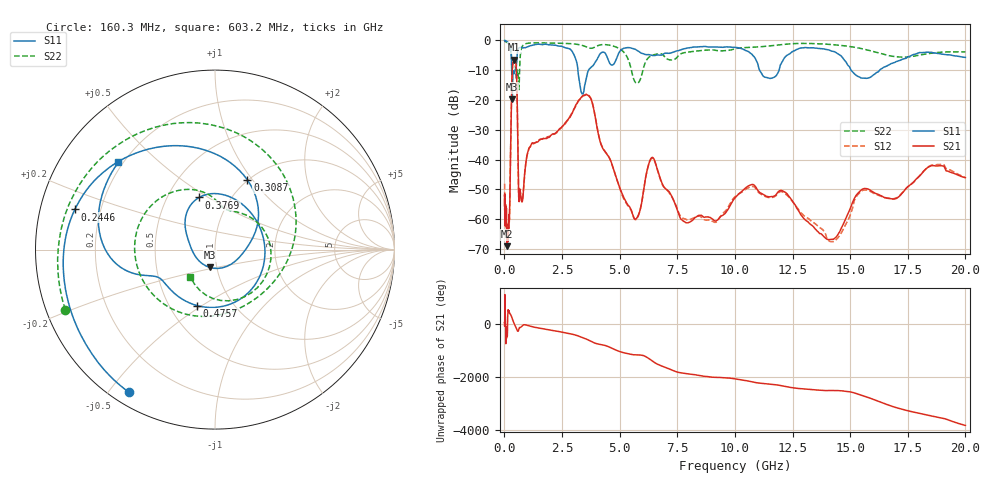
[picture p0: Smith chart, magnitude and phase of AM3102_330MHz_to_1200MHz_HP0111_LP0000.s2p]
! Date/Time: Tue, Sep 11, 2018 5:15 PM
! Network Analyzer: Agilent Technologies E8362B Rev: A.07.50.63
! Sweep from 0.010 to 20.000 GHz, 1601 Points, Sweep Type: LOG
! Power Supply: 4.949 V, 0.001 A
# Hz S DB R 50
!freq MagS11 AngS11 MagS21 AngS21 MagS12 AngS12 MagS22 AngS22
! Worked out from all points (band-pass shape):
!   1601 points, 10 MHz to 20 GHz, reference 50 ohm
!   highest |S21| = -6.39 dB at 424.4 MHz (marker M1); lowest = -69.0 dB at 112.2 MHz (marker M2)
!   |S21| within 3 dB of the highest: 344.1 MHz to 517.9 MHz (173.8 MHz wide, 40.3 % of centre)
!   lowest |S11| = -19.7 dB at 341.1 MHz (marker M3), VSWR 1.23, Z = 46.2 - j9.27 ohm
!   |S11| at or under -10 dB: 3.19 GHz to 3.649 GHz (458.7 MHz wide, 13.4 % of centre); 11.08 GHz to 11.92 GHz (840 MHz wide, 7.31 % of centre); 15.04 GHz to 16.28 GHz (1.233 GHz wide, 7.88 % of centre)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
!   |S22| runs from -16.5 to -0.2 dB; largest |S21 - S12| = 0.0058
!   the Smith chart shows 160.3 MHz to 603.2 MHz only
!   S11 on the Smith chart (normalised r, x): 160.3 MHz: 0.05, -0.56; 244.6 MHz: 0.11, +0.14; 308.7 MHz: 0.99, +0.94; 376.9 MHz: 0.72, +0.46; 475.7 MHz: 0.68, -0.48; 603.2 MHz: 0.18, +0.37
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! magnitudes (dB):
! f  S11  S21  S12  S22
! 10 MHz  0.0  -53.2  -48.1  -0.2
! 35.55 MHz  0.0  -60.0  -60.0  -0.3
! 112.2 MHz  -0.3  -69.0  -63.6  -0.6
! 126.4 MHz  -0.4  -63.6  -66.0  -0.7
! 160.3 MHz  -0.6  -65.0  -66.7  -0.9
! 244.6 MHz  -1.8  -50.3  -49.9  -2.0
! 308.7 MHz  -7.4  -19.1  -19.2  -5.2
! 341.1 MHz  -19.7  -9.8  -9.9  -8.7
! 376.9 MHz  -10.3  -7.1  -7.2  -8.2
! 424.4 MHz  -11.1  -6.4  -6.4  -7.0
! 447.2 MHz  -10.4  -6.5  -6.5  -7.1
! 475.7 MHz  -9.7  -6.8  -6.8  -8.4
! 603.2 MHz  -2.8  -45.7  -45.1  -13.8
! 772.3 MHz  -2.5  -54.1  -53.8  -2.0
! 1.59 GHz  -1.4  -33.1  -33.1  -0.8
! 3.617 GHz  -10.6  -18.4  -18.1  -2.4
! 5.652 GHz  -2.9  -59.9  -60.0  -13.7
! 6.426 GHz  -5.0  -39.2  -39.6  -4.9
! 7.845 GHz  -2.7  -61.0  -59.9  -4.0
! 10.73 GHz  -4.6  -48.3  -49.0  -2.3
! 14.21 GHz  -3.6  -66.7  -67.5  -1.4
! 20 GHz  -5.7  -46.0  -46.0  -3.8
